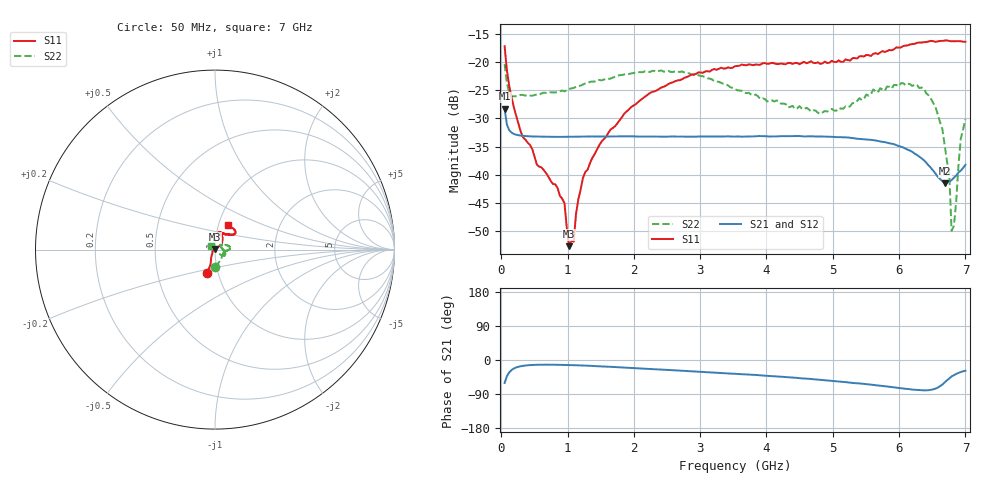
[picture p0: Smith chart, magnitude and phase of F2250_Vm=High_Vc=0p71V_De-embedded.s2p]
! Integrated Device Technology
! Corporate Headquarters
! 6024 Silver Creek Valley Road
! San Jose, CA 95138  USA
! Phone:  1-408-284-8200
! Toll Free:  1-800-223-1366
! Webpage:  http://www.idt.com/
! Timing and RF Division
! 515 Groton Road, Suite 102
! Westford, MA 01886-6024
! Device:  F2250
! Description: Voltage Variable RF Attenuator
! Frequency:  50.0 -  6000.00 MHz
! Package:  3x3 mm Thin QFN Plastic Package: 16 pin
! Ports:  2 RF, 3 DC
!  Pin  1  = GND
!  Pin  2  = NC
!  Pin  3  = RF1  = Port 1
!  Pin  4  = NC
!  Pin  5  = GND
!  Pin  6  = GND
!  Pin  7  = GND
!  Pin  8  = GND
!  Pin  9  = NC
!  Pin 10  = RF2  = Port 2
!  Pin 11  = NC
!  Pin 12  = GND
!  Pin 13  = GND
!  Pin 14  = VCNTRL
!  Pin 15  = VDD
!  Pin 16  = VMODE
! Vcntrl:  0.710 Volts
! Vmode:  +3.300 Volts
! Vdd:  +3.30  Volts
! Current:  1.293 mA
! Data:  The device was measured on a the F2250 evaluation board which has
!  individual transmission lines to the RF pins.  Data was collected
!  using a calibrated network analyzer.  The evaluation board was
!  de-embedded using a TRL calibration technique.
!  The reference plane is the edge of the package pin.
! Misc:  SN 10
!  Action Tracker AT0258
! Date Measured:  2014-11-26
! Date:  2015-10-15  MJV
! Note:
!  Integrated Device Technology supplies this data as a sample of measured
!  data at the package pin for this product.  Your particular data for this
!  product may vary.
!  Data was taken at 25 degrees C.
!  Integrated Device Technology reserves the right to change this data at anytime.
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# GHz S dB R 50
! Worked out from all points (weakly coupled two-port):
!   201 points, 50 MHz to 7 GHz, reference 50 ohm
!   highest |S21| = -28.28 dB at 50 MHz (marker M1); lowest = -41.5 dB at 6.687 GHz (marker M2)
!   lowest |S11| = -52.7 dB at 1.023 GHz (marker M3), VSWR 1.00, Z = 49.8 + j0.161 ohm
!   |S11| at or under -10 dB: start of sweep to end of sweep
!   |S22| runs from -50.0 to -20.3 dB; largest |S21 - S12| = 7e-05
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0.05  -17.16 -108.1  -28.28 -60.4  -28.27 -60.4  -20.32 -88.8
0.1195  -24.20 -111.3  -32.08 -32.6  -32.08 -32.5  -25.31 -43.8
0.29325  -32.35 -126.0  -33.06 -16.4  -33.06 -16.4  -25.80 -18.6
0.9535  -45.11 171.7  -33.28 -13.0  -33.28 -13.0  -25.16 -7.0
1.023  -52.73 135.6  -33.27 -13.3  -33.27 -13.3  -24.74 -6.4
1.0925  -51.92 77.1  -33.26 -13.6  -33.27 -13.7  -24.57 -5.8
1.12725  -46.97 53.6  -33.26 -13.9  -33.26 -13.9  -24.36 -6.3
1.2315  -40.60 37.5  -33.24 -14.5  -33.25 -14.5  -23.96 -6.9
1.6485  -31.96 39.8  -33.21 -18.0  -33.21 -18.0  -22.90 -2.6
2.37825  -24.75 46.1  -33.23 -25.0  -33.23 -25.0  -21.55 5.3
3.525  -20.69 71.4  -33.23 -36.3  -33.23 -36.4  -24.73 26.1
4.7065  -20.10 71.8  -33.18 -50.7  -33.19 -50.7  -28.56 32.1
5.15825  -19.93 56.2  -33.36 -57.6  -33.35 -57.6  -28.26 10.2
5.85325  -17.81 40.4  -34.42 -70.6  -34.41 -70.8  -24.37 -18.6
6.3745  -16.42 40.8  -37.44 -80.0  -37.43 -80.1  -24.71 -34.7
6.54825  -16.36 44.5  -39.80 -75.6  -39.81 -75.6  -27.94 -43.7
6.68725  -16.13 47.7  -41.55 -59.4  -41.52 -59.5  -34.69 -43.5
6.75675  -16.21 50.4  -41.22 -48.9  -41.21 -48.9  -39.65 -51.9
6.7915  -16.27 51.2  -40.99 -43.4  -40.97 -43.4  -50.00 -26.8
6.82625  -16.25 52.4  -40.55 -39.9  -40.51 -40.1  -49.15 163.3
6.9305  -16.25 58.6  -39.28 -31.9  -39.26 -32.0  -33.58 136.8
7  -16.36 62.3  -38.25 -28.4  -38.24 -28.2  -30.14 134.9
